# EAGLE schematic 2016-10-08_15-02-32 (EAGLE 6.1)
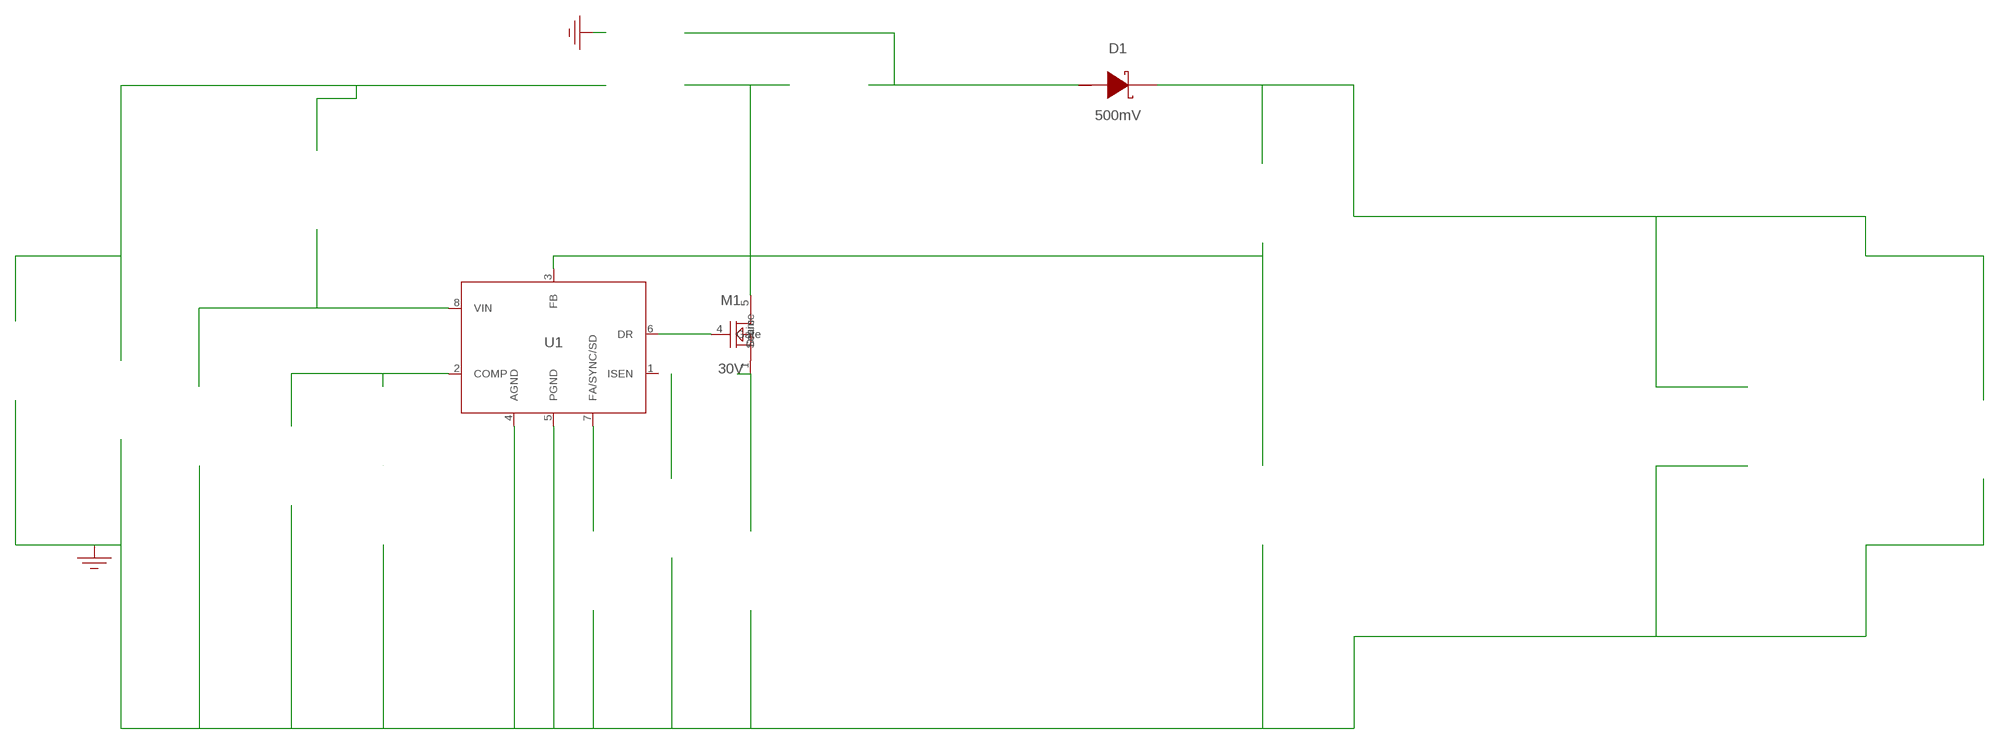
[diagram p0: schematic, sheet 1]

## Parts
CBP  100nF  GRM155R61A104KA01DGRM155R61A104KA01D  [0402]  (not placed on a sheet)
CCOMP  82nF  GRM155R61A823KA01DGRM155R61A823KA01D  [0402]  (not placed on a sheet)
CCOMP2  5.1nF  GRM2195C1H512JA01DGRM2195C1H512JA01D  [0805]  (not placed on a sheet)
CIN  4.7uF  10TPU4R7MSI10TPU4R7MSI  [CAPSMT_6_S09]  (not placed on a sheet)
COUT  100uF  GRM31CR60J107ME39LGRM31CR60J107ME39L  [1206_190]  (not placed on a sheet)
COUT_2  100uF  GRM31CR60J107ME39LGRM31CR60J107ME39L  [1206_190]  (not placed on a sheet)
CRAMP  1.2nF  CL21C122JBFNNWECL21C122JBFNNWE  [0805]  (not placed on a sheet)
CSEP  2.2uF  GRM21BR71A225KA01LGRM21BR71A225KA01L  [0805]  (not placed on a sheet)
D1  500mV  B220-13-FB220-13-F  [SMB]
GND  WB_GND  WB_GNDWB_GND  [WB_GND]
GND100  WB_GND  WB_GNDWB_GND  [WB_GND]
IOUT  WB_CURRENT_LOAD  WB_CURRENT_LOADWB_CURRENT_LOAD  [WB_CURRENT_LOAD]  (not placed on a sheet)
LIN  12uH  NPI75C120MTRFNPI75C120MTRF  [IND_NPI75C]  (not placed on a sheet)
LOUT  33uH  SRN8040-330MSRN8040-330M  [SRN8040]  (not placed on a sheet)
M1  30V  CSD17308Q3CSD17308Q3  [DQG0008A]
RBP  20  CRCW040220R0FKEDCRCW040220R0FKED  [0402]  (not placed on a sheet)
RCOMP  1.18k  CRCW04021K18FKEDCRCW04021K18FKED  [0402]  (not placed on a sheet)
RFADJ  69.8k  CRCW040269K8FKEDCRCW040269K8FKED  [0402]  (not placed on a sheet)
RFB1  10k  CRCW040210K0FKEDCRCW040210K0FKED  [0402]  (not placed on a sheet)
RFB2  16.2k  CRCW040216K2FKEDCRCW040216K2FKED  [0402]  (not placed on a sheet)
RRAMP  100  CRCW0402100RFKEDCRCW0402100RFKED  [0402]  (not placed on a sheet)
RSENSE  33m  ERJ-L14KF33MUERJ-L14KF33MU  [1210]  (not placed on a sheet)
U1  LM3488MMX/NOPB  LM3488MMX/NOPBLM3488MMX/NOPB  [MUA08A]
VIN  WB_BATTERY  WB_BATTERYWB_BATTERY  [WB_BATTERY]  (not placed on a sheet)

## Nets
0: Cbp.2@2 Ccomp2.2@2 Ccomp.2@2 Cin.-@2 Cout.2@2 Cout_2.2@2 Cramp.2@2 GND100.1 GND.1 Iout.-@2 Lout.2@2 Rfadj.1@1 Rfb1.2@2 Rsense.2@2 U1.4(AGND) U1.5(PGND) Vin.-@2
1: Rfadj.2@2 U1.7(FA/SYNC/SD)
2: Cout.1@1 Cout_2.1@1 D1.1(K) Iout.+@1 Rfb2.1@1
3: Cin.+@1 Lin.2@2 Rbp.1@1 Vin.+@1
4: Ccomp2.1@1 Rcomp.1@1 U1.2(COMP)
5: Csep.1@1 D1.2(A) Lout.1@1
6: Cramp.1@1
7: Cbp.1@1 Rbp.2@2 U1.8(VIN)
8: Rfb1.1@1 Rfb2.2@2 U1.3(FB)
9: M1.1(Source) M1.2(Source) M1.3(Source) Rramp.2@2 Rsense.1@1
10: Csep.2@2 Lin.1@1 M1.5(Drain) M1.6(Drain) M1.7(Drain) M1.8(Drain) M1.9(Drain)
11: M1.4(Gate) U1.6(DR)
12: Rramp.1@1 U1.1(ISEN)
13: Ccomp.1@1 Rcomp.2@2
Unconnected: CBP.1 CBP.2 CCOMP2.1 CCOMP2.2 CCOMP.1 CCOMP.2 CIN.1(+) CIN.2(-) COUT.1 COUT.2 COUT_2.1 COUT_2.2 CRAMP.1 CRAMP.2 CSEP.1 CSEP.2 IOUT.1(+) IOUT.2(-) LIN.1 LIN.2 LOUT.1 LOUT.2 RBP.1 RBP.2 RCOMP.1 RCOMP.2 RFADJ.1 RFADJ.2 RFB1.1 RFB1.2 RFB2.1 RFB2.2 RRAMP.1 RRAMP.2 RSENSE.1 RSENSE.2 VIN.1(+) VIN.2(-)

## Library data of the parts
CBP = AcceleratedDesigns_Lib:GRM155R61A104KA01D; Cap: 1.0E-7; ESR: 0.0; IRMS: 0.0; Manufacturer_Name: MuRata; Manufacturer_Part_Number: GRM155R61A104KA01D; VDC: 10.0; Vendor: MuRata
CCOMP = AcceleratedDesigns_Lib:GRM155R61A823KA01D; Cap: 8.2E-8; ESR: 0.0; IRMS: 0.0; Manufacturer_Name: MuRata; Manufacturer_Part_Number: GRM155R61A823KA01D; VDC: 10.0; Vendor: MuRata
CCOMP2 = AcceleratedDesigns_Lib:GRM2195C1H512JA01D; Cap: 5.1E-9; ESR: 0.0; IRMS: 0.0; Manufacturer_Name: MuRata; Manufacturer_Part_Number: GRM2195C1H512JA01D; VDC: 50.0; Vendor: MuRata
CIN = AcceleratedDesigns_Lib:10TPU4R7MSI; Cap: 4.7E-6; Datasheet_URL: http://industrial.panasonic.com/www%2Ddata/pdf/AAA8000/AAA8000CE1.pdf; ESR: 0.3; IRMS: 0.36; Manufacturer_Name: Panasonic; Manufacturer_Part_Number: 10TPU4R7MSI; VDC: 10.0; Vendor: Panasonic
COUT COUT_2 = AcceleratedDesigns_Lib:GRM31CR60J107ME39L; Cap: 1.0E-4; ESR: 0.0030; IRMS: 0.0; Manufacturer_Name: MuRata; Manufacturer_Part_Number: GRM31CR60J107ME39L; VDC: 6.3; Vendor: MuRata
CRAMP = AcceleratedDesigns_Lib:CL21C122JBFNNWE; Cap: 1.2E-9; Datasheet_URL: http://www.samsungsem.com/servlet/FileDownload?type%3Dspec%26file%3DCL21C122JBFNNWE.pdf; ESR: 0.0; IRMS: 0.0; Manufacturer_Name: Samsung Electro-Mechanics; Manufacturer_Part_Number: CL21C122JBFNNWE; VDC: 50.0; Vendor: Samsung Electro-Mechanics
CSEP = AcceleratedDesigns_Lib:GRM21BR71A225KA01L; Cap: 2.2E-6; ESR: 0.0060; IRMS: 0.0; Manufacturer_Name: MuRata; Manufacturer_Part_Number: GRM21BR71A225KA01L; VDC: 10.0; Vendor: MuRata
D1 = AcceleratedDesigns_Lib:B220-13-F; Datasheet_URL: http://www.diodes.com/datasheets/ds13004.pdf; Io: 2.0; Manufacturer_Name: Diodes Inc.; Manufacturer_Part_Number: B220-13-F; VFatIo: 0.5; VRRM: 20.0; Vendor: Diodes Inc.
GND GND100 = AcceleratedDesigns_Lib:WB_GND; Manufacturer_Name: WB_GND; Manufacturer_Part_Number: WB_GND; PowerPortType: POWER_GROUND; Value: Value
IOUT = AcceleratedDesigns_Lib:WB_CURRENT_LOAD; Manufacturer_Name: WB_CURRENT_LOAD; Manufacturer_Part_Number: WB_CURRENT_LOAD; PowerPortType: POWER_GROUND; Value: Value
LIN = AcceleratedDesigns_Lib:NPI75C120MTRF; DCR: 0.08; IDC: 2.0; L: 1.2E-5; Manufacturer_Name: NIC Components; Manufacturer_Part_Number: NPI75C120MTRF; Vendor: NIC Components
LOUT = AcceleratedDesigns_Lib:SRN8040-330M; DCR: 0.145; Datasheet_URL: http://www.bourns.com/data/global/pdfs/SRN8040.pdf; IDC: 1.7; L: 3.3E-5; Manufacturer_Name: Bourns; Manufacturer_Part_Number: SRN8040-330M; Vendor: Bourns
M1 = AcceleratedDesigns_Lib:CSD17308Q3; Datasheet_URL: http://www.ti.com/lit/ds/symlink/csd17308q3.pdf; IdsMax: 50.0; Manufacturer_Name: Texas Instruments; Manufacturer_Part_Number: CSD17308Q3; QgTyp: 3.9; Quantity: 1; Rdson45: 0.0094; VdsMax: 30.0; Vendor: Texas Instruments
RBP = AcceleratedDesigns_Lib:CRCW040220R0FKED; Manufacturer_Name: Vishay-Dale; Manufacturer_Part_Number: CRCW040220R0FKED; Power: 0.063; Resistance: 20.0; Tolerance: 1.0; Vendor: Vishay-Dale
RCOMP = AcceleratedDesigns_Lib:CRCW04021K18FKED; Manufacturer_Name: Vishay-Dale; Manufacturer_Part_Number: CRCW04021K18FKED; Power: 0.063; Resistance: 1180.0; Tolerance: 1.0; Vendor: Vishay-Dale
RFADJ = AcceleratedDesigns_Lib:CRCW040269K8FKED; Manufacturer_Name: Vishay-Dale; Manufacturer_Part_Number: CRCW040269K8FKED; Power: 0.063; Resistance: 69800.0; Tolerance: 1.0; Vendor: Vishay-Dale
RFB1 = AcceleratedDesigns_Lib:CRCW040210K0FKED; Manufacturer_Name: Vishay-Dale; Manufacturer_Part_Number: CRCW040210K0FKED; Power: 0.063; Resistance: 10000.0; Tolerance: 1.0; Vendor: Vishay-Dale
RFB2 = AcceleratedDesigns_Lib:CRCW040216K2FKED; Manufacturer_Name: Vishay-Dale; Manufacturer_Part_Number: CRCW040216K2FKED; Power: 0.063; Resistance: 16200.0; Tolerance: 1.0; Vendor: Vishay-Dale
RRAMP = AcceleratedDesigns_Lib:CRCW0402100RFKED; Manufacturer_Name: Vishay-Dale; Manufacturer_Part_Number: CRCW0402100RFKED; Power: 0.063; Resistance: 100.0; Tolerance: 1.0; Vendor: Vishay-Dale
RSENSE = AcceleratedDesigns_Lib:ERJ-L14KF33MU; Manufacturer_Name: Panasonic; Manufacturer_Part_Number: ERJ-L14KF33MU; Power: 0.33; Resistance: 0.033; Tolerance: 1.0; Vendor: Panasonic
U1 = AcceleratedDesigns_Lib:LM3488MMX/NOPB; Datasheet_URL: http://www.ti.com/product/lm3488; Frequency: 1000000.0; Imax: 20.0; Manufacturer_Name: Texas Instruments; Manufacturer_Part_Number: LM3488MM/NOPB; Mktg_Package: NA; NSID: LM3488MM/NOPB; Package: NA; Vendor: Texas Instruments
VIN = AcceleratedDesigns_Lib:WB_BATTERY; Manufacturer_Name: WB_BATTERY; Manufacturer_Part_Number: WB_BATTERY; PowerPortType: POWER_GROUND; Value: Value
